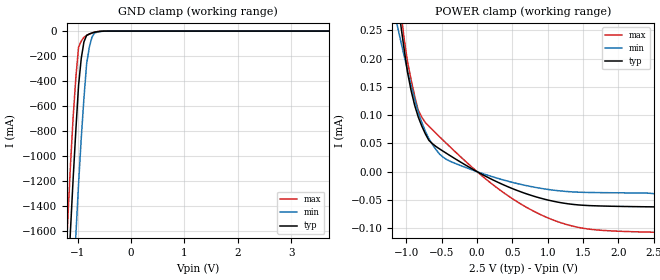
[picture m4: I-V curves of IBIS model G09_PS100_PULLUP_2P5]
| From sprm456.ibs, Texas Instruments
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|IDG09_PS100_NOPULLUP_2P75; BUFFER OPERATING IN NORMMAL MODE WITHOUT PULLUP
|   Model Cell G09_PS100_PULLUP_2P5
|IDG09_PS100_PULLUP_2P5
[Model]   G09_PS100_PULLUP_2P5
Model_type   Input
Polarity   Non-Inverting
Vinl =  0.7V
Vinh =  1.7V
C_comp   1.242p   1.179p   1.348p
[Model Spec]
Vinl   0.7V   0.7V   0.7V
Vinh   1.7V   1.7V   1.7V
[Temperature Range]   25   125   -40
[Voltage Range]   2.5   2.3   2.7
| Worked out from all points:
|   GND clamp passes 1 mA (typ) near -0.54 V on its own axis
|   POWER clamp passes 1 mA (typ) near -1.78 V on its own axis
[POWER_clamp]
|   voltage   I(typ)   I(min)   I(max)
-2.5V     1.8mA      1.08mA     2.671mA
-1.136V   313.2uA    262.1uA    357.3uA
-1.086V   264.7uA    233.8uA    291.9uA
-1.035V   218.8uA    206.1uA    237.5uA
-934.3mV  143.7uA    152.9uA    162.6uA
-782.8mV  80.61uA    87uA       96.3uA
-580.8mV  44.38uA    38.8uA     67.78uA
-378.8mV  28.1uA     18.2uA     43.38uA
328.3mV   -20.7uA    -13.1uA    -32.87uA
984.8mV   -49.63uA   -31.07uA   -80.85uA
1.591V    -60uA      -36.78uA   -101.7uA
2.5V      -62.22uA   -38.9uA    -107.1uA
[GND_clamp]
|   voltage   I(typ)   I(min)   I(max)
-2.5V     -14.65A    -15.5A     -14.18A
-1.237V   -2.489A    -3.395A    -1.958A
-1.187V   -2.038A    -2.94A     -1.511A
-1.136V   -1.594A    -2.491A    -1.074A
-1.035V   -791.1mA   -1.633A    -371.5mA
-984.8mV  -434.4mA   -1.223A    -129.4mA
-934.3mV  -219.3mA   -857.5mA   -80.06mA
-833.3mV  -33.77mA   -260.3mA   -35.39mA
-782.8mV  -23mA      -128.3mA   -24.98mA
-681.8mV  -8.417mA   -15mA      -8.191mA
-530.3mV  -652.7uA   -1.553mA   -364.1uA
5V        0A         0A         0A
